| IBIS file stm32l0_71_72_73_81_82_83_wlcsp49.ibs
| Created by s2ibis version 1.1 (customized version)
| North Carolina State University, ERL, 2006
[IBIS ver] 4.2
[File name] stm32l0_71_72_73_81_82_83_wlcsp49.ibs
[File Rev] 1.0
[Date]  14-03-2016
[Source] Data Created at STMicroelectronics
[Notes]  File originated from ELDO simulations.
[Disclaimer]  This information is for modeling purpose only and is
   not guaranted. The information is subject to change without
   notice.
[Copyright] Copyright 2016 STMicroelectronics Inc.
|   Component stm32l0_71_72_73_81_82_83_wlcsp49
[Component] stm32l0_71_72_73_81_82_83_wlcsp49
[Manufacturer] STMicroelectronics
[Package]
| variable   typ   min   max
R_pkg   0.0   0.0   0.0
L_pkg   0.0H   0.0H   0.0H
C_pkg   0.0F   0.0F   0.0F
[Pin]  signal_name   model_name   R_pin   L_pin   C_pin
B6 VLCD POWER
B7 PC13 io8p_wsudq_ls_ft_v33
C6 PC14-OSC32_IN io8p_wsudq_ls_ft_v33
C7 PC15-OSC32_OUT io8p_sudq_ls_tc_esdft
D6 PH0-OSC_IN io8p_sudq_ls_tc_esdft
D7 PH1-OSC_OUT io8p_sudq_ls_tc_esdft
D5 NRST ioreset_ft_v33
C5 PC0 io8p_sudq_lcd4_i2cin_ls_ft
C4 PC1 io8p_sudq_lcd4_i2cin_ls_ft
E7 PC2 io8p_wsudq_lcd4_ls_ft
E6 VREF+ POWER
F7 VDDA POWER
E5 PA0 io8p_wsudq_ls_ft_v33
E4 PA1 io8p_wsudq_lcd4_ls_ft
F6 PA2 io8p_wsudq_lcd4_ls_ft
G7 PA3 io8p_wsudq_lcd4_ls_ft
F5 PA4 io8p_wsudq_i2cin_ls_ft
G6 PA5 io8p_wsudq_i2cin_ls_ft
G5 PA6 io8p_wsudq_lcd4_ls_ft
F4 PA7 io8p_wsudq_lcd4_ls_ft
G4 PB0 io8p_wsudq_lcd4_ls_ft
D3 PB1 io8p_wsudq_lcd4_ls_ft
E3 PB2 io8p_wsudq_lcd4_ls_ft
G3 PB10 io8p_sudq_lcd4_i2cin_ls_ft
F3 PB11 io8p_sudq_lcd4_i2cin_ls_ft
D4 VSS GND
G2 VDD POWER
G1 PB12 io8p_wsudq_lcd4_ls_ft
F2 PB13 io8p_sudq_lcd4_i2cin_ls_ft
F1 PB14 io8p_sudq_lcd4_i2cin_ls_ft
E1 PB15 io8p_wsudq_lcd4_ls_ft
D1 PA8 io8p_sudq_lcd4_i2cin_ls_ft
E2 PA9 io8p_sudq_lcd4_i2cin_ls_ft
C1 PA10 io8p_sudq_lcd4_i2cin_ls_ft
D2 PA11 io8usb_ls_ft
B1 PA12 io8usb_ls_ft
C2 PA13 io8p_sudq_ls_ft
A1 VDD_USB POWER
B2 PA14 io8p_sudq_ls_ft
A2 PA15 io8p_wsudq_lcd4_ls_ft
A3 PB3 io8p_wsudq_lcd4_ls_ft
B3 PB4 io8p_sudq_lcd4_i2cin_ls_ft
A4 PB5 io8p_wsudq_lcd4_ls_ft
B4 PB6 io8p_wsudq_i2cin_ls_ft
C3 PB7 io8p_wsudq_i2cin_ls_ft
A5 BOOT0 vpp_test_hv
B5 PB8 io8p_sudq_lcd4_i2cin_ls_ft
A6 PB9 io8p_sudq_lcd4_i2cin_ls_ft
A7 VDD POWER
[Model Selector] io8p_sudq_ls_ft
io8p00_sudq_ls_ft_pd_lv  "SPEED00 1P8V, PD=40kOhm"
io8p00_sudq_ls_ft_pu_lv  "SPEED00 1P8V, PU=40kOhm"
io8p00_sudq_ls_ft_lv  "SPEED00 1P8V"
io8p01_sudq_ls_ft_pd_lv  "SPEED01 1P8V, PD=40kOhm"
io8p01_sudq_ls_ft_pu_lv  "SPEED01 1P8V, PU=40kOhm"
io8p01_sudq_ls_ft_lv  "SPEED01 1P8V"
io8p10_sudq_ls_ft_pd_lv  "SPEED10 1P8V, PD=40kOhm"
io8p10_sudq_ls_ft_pu_lv  "SPEED10 1P8V, PU=40kOhm"
io8p10_sudq_ls_ft_lv  "SPEED10 1P8V"
io8p11_sudq_ls_ft_pd_lv  "SPEED11 1P8V, PD=40kOhm"
io8p11_sudq_ls_ft_pu_lv  "SPEED11 1P8V, PU=40kOhm"
io8p11_sudq_ls_ft_lv  "SPEED11 1P8V"
io8p00_sudq_ls_ft_pd  "SPEED00, PD=40kOhm"
io8p00_sudq_ls_ft_pu  "SPEED00, PU=40kOhm"
io8p00_sudq_ls_ft  "SPEED00"
io8p01_sudq_ls_ft_pd  "SPEED01, PD=40kOhm"
io8p01_sudq_ls_ft_pu  "SPEED01, PU=40kOhm"
io8p01_sudq_ls_ft  "SPEED01"
io8p10_sudq_ls_ft_pd  "SPEED10, PD=40kOhm"
io8p10_sudq_ls_ft_pu  "SPEED10, PU=40kOhm"
io8p10_sudq_ls_ft  "SPEED10"
io8p11_sudq_ls_ft_pd  "SPEED11, PD=40kOhm"
io8p11_sudq_ls_ft_pu  "SPEED11, PU=40kOhm"
io8p11_sudq_ls_ft  "SPEED11"
[Model Selector] io8p_sudq_ls_tc_esdft
io8p00_sudq_ls_tc_esdft_pd_lv  "SPEED00 1P8V, PD=40kOhm"
io8p00_sudq_ls_tc_esdft_pu_lv  "SPEED00 1P8V, PU=40kOhm"
io8p00_sudq_ls_tc_esdft_lv  "SPEED00 1P8V"
io8p01_sudq_ls_tc_esdft_pd_lv  "SPEED01 1P8V, PD=40kOhm"
io8p01_sudq_ls_tc_esdft_pu_lv  "SPEED01 1P8V, PU=40kOhm"
io8p01_sudq_ls_tc_esdft_lv  "SPEED01 1P8V"
io8p10_sudq_ls_tc_esdft_pd_lv  "SPEED10 1P8V, PD=40kOhm"
io8p10_sudq_ls_tc_esdft_pu_lv  "SPEED10 1P8V, PU=40kOhm"
io8p10_sudq_ls_tc_esdft_lv  "SPEED10 1P8V"
io8p11_sudq_ls_tc_esdft_pd_lv  "SPEED11 1P8V, PD=40kOhm"
io8p11_sudq_ls_tc_esdft_pu_lv  "SPEED11 1P8V, PU=40kOhm"
io8p11_sudq_ls_tc_esdft_lv  "SPEED11 1P8V"
io8p00_sudq_ls_tc_esdft_pd  "SPEED00, PD=40kOhm"
io8p00_sudq_ls_tc_esdft_pu  "SPEED00, PU=40kOhm"
io8p00_sudq_ls_tc_esdft  "SPEED00"
io8p01_sudq_ls_tc_esdft_pd  "SPEED01, PD=40kOhm"
io8p01_sudq_ls_tc_esdft_pu  "SPEED01, PU=40kOhm"
io8p01_sudq_ls_tc_esdft  "SPEED01"
io8p10_sudq_ls_tc_esdft_pd  "SPEED10, PD=40kOhm"
io8p10_sudq_ls_tc_esdft_pu  "SPEED10, PU=40kOhm"
io8p10_sudq_ls_tc_esdft  "SPEED10"
io8p11_sudq_ls_tc_esdft_pd  "SPEED11, PD=40kOhm"
io8p11_sudq_ls_tc_esdft_pu  "SPEED11, PU=40kOhm"
io8p11_sudq_ls_tc_esdft  "SPEED11"
[Model Selector] io8p_wsudq_i2cin_ls_ft
io8p00_wsudq_i2cin_ls_ft_pd_lv  "SPEED00 1P8V, PD=40kOhm"
io8p00_wsudq_i2cin_ls_ft_pu_lv  "SPEED00 1P8V, PU=40kOhm"
io8p00_wsudq_i2cin_ls_ft_lv  "SPEED00 1P8V"
io8p01_wsudq_i2cin_ls_ft_pd_lv  "SPEED01 1P8V, PD=40kOhm"
io8p01_wsudq_i2cin_ls_ft_pu_lv  "SPEED01 1P8V, PU=40kOhm"
io8p01_wsudq_i2cin_ls_ft_lv  "SPEED01 1P8V"
io8p10_wsudq_i2cin_ls_ft_pd_lv  "SPEED10 1P8V, PD=40kOhm"
io8p10_wsudq_i2cin_ls_ft_pu_lv  "SPEED10 1P8V, PU=40kOhm"
io8p10_wsudq_i2cin_ls_ft_lv  "SPEED10 1P8V"
io8p11_wsudq_i2cin_ls_ft_pd_lv  "SPEED11 1P8V, PD=40kOhm"
io8p11_wsudq_i2cin_ls_ft_pu_lv  "SPEED11 1P8V, PU=40kOhm"
io8p11_wsudq_i2cin_ls_ft_lv  "SPEED11 1P8V"
io8p00_wsudq_i2cin_ls_ft_pd  "SPEED00, PD=40kOhm"
io8p00_wsudq_i2cin_ls_ft_pu  "SPEED00, PU=40kOhm"
io8p00_wsudq_i2cin_ls_ft  "SPEED00"
io8p01_wsudq_i2cin_ls_ft_pd  "SPEED01, PD=40kOhm"
io8p01_wsudq_i2cin_ls_ft_pu  "SPEED01, PU=40kOhm"
io8p01_wsudq_i2cin_ls_ft  "SPEED01"
io8p10_wsudq_i2cin_ls_ft_pd  "SPEED10, PD=40kOhm"
io8p10_wsudq_i2cin_ls_ft_pu  "SPEED10, PU=40kOhm"
io8p10_wsudq_i2cin_ls_ft  "SPEED10"
io8p11_wsudq_i2cin_ls_ft_pd  "SPEED11, PD=40kOhm"
io8p11_wsudq_i2cin_ls_ft_pu  "SPEED11, PU=40kOhm"
io8p11_wsudq_i2cin_ls_ft  "SPEED11"
[Model Selector] io8p_wsudq_lcd4_ls_ft
io8p00_wsudq_lcd4_ls_ft_pd_lv  "SPEED00 1P8V, PD=40kOhm"
io8p00_wsudq_lcd4_ls_ft_pu_lv  "SPEED00 1P8V, PU=40kOhm"
io8p00_wsudq_lcd4_ls_ft_lv  "SPEED00 1P8V"
io8p01_wsudq_lcd4_ls_ft_pd_lv  "SPEED01 1P8V, PD=40kOhm"
io8p01_wsudq_lcd4_ls_ft_pu_lv  "SPEED01 1P8V, PU=40kOhm"
io8p01_wsudq_lcd4_ls_ft_lv  "SPEED01 1P8V"
io8p10_wsudq_lcd4_ls_ft_pd_lv  "SPEED10 1P8V, PD=40kOhm"
io8p10_wsudq_lcd4_ls_ft_pu_lv  "SPEED10 1P8V, PU=40kOhm"
io8p10_wsudq_lcd4_ls_ft_lv  "SPEED10 1P8V"
io8p11_wsudq_lcd4_ls_ft_pd_lv  "SPEED11 1P8V, PD=40kOhm"
io8p11_wsudq_lcd4_ls_ft_pu_lv  "SPEED11 1P8V, PU=40kOhm"
io8p11_wsudq_lcd4_ls_ft_lv  "SPEED11 1P8V"
io8p00_wsudq_lcd4_ls_ft_pd  "SPEED00, PD=40kOhm"
io8p00_wsudq_lcd4_ls_ft_pu  "SPEED00, PU=40kOhm"
io8p00_wsudq_lcd4_ls_ft  "SPEED00"
io8p01_wsudq_lcd4_ls_ft_pd  "SPEED01, PD=40kOhm"
io8p01_wsudq_lcd4_ls_ft_pu  "SPEED01, PU=40kOhm"
io8p01_wsudq_lcd4_ls_ft  "SPEED01"
io8p10_wsudq_lcd4_ls_ft_pd  "SPEED10, PD=40kOhm"
io8p10_wsudq_lcd4_ls_ft_pu  "SPEED10, PU=40kOhm"
io8p10_wsudq_lcd4_ls_ft  "SPEED10"
io8p11_wsudq_lcd4_ls_ft_pd  "SPEED11, PD=40kOhm"
io8p11_wsudq_lcd4_ls_ft_pu  "SPEED11, PU=40kOhm"
io8p11_wsudq_lcd4_ls_ft  "SPEED11"
[Model Selector] io8p_wsudq_ls_ft_v33
io8p00_wsudq_ls_ft_v33_pd_lv  "SPEED00 1P8V, PD=40kOhm"
io8p00_wsudq_ls_ft_v33_pu_lv  "SPEED00 1P8V, PU=40kOhm"
io8p00_wsudq_ls_ft_v33_lv  "SPEED00 1P8V"
io8p01_wsudq_ls_ft_v33_pd_lv  "SPEED01 1P8V, PD=40kOhm"
io8p01_wsudq_ls_ft_v33_pu_lv  "SPEED01 1P8V, PU=40kOhm"
io8p01_wsudq_ls_ft_v33_lv  "SPEED01 1P8V"
io8p10_wsudq_ls_ft_v33_pd_lv  "SPEED10 1P8V, PD=40kOhm"
io8p10_wsudq_ls_ft_v33_pu_lv  "SPEED10 1P8V, PU=40kOhm"
io8p10_wsudq_ls_ft_v33_lv  "SPEED10 1P8V"
io8p11_wsudq_ls_ft_v33_pd_lv  "SPEED11 1P8V, PD=40kOhm"
io8p11_wsudq_ls_ft_v33_pu_lv  "SPEED11 1P8V, PU=40kOhm"
io8p11_wsudq_ls_ft_v33_lv  "SPEED11 1P8V"
io8p00_wsudq_ls_ft_v33_pd  "SPEED00, PD=40kOhm"
io8p00_wsudq_ls_ft_v33_pu  "SPEED00, PU=40kOhm"
io8p00_wsudq_ls_ft_v33  "SPEED00"
io8p01_wsudq_ls_ft_v33_pd  "SPEED01, PD=40kOhm"
io8p01_wsudq_ls_ft_v33_pu  "SPEED01, PU=40kOhm"
io8p01_wsudq_ls_ft_v33  "SPEED01"
io8p10_wsudq_ls_ft_v33_pd  "SPEED10, PD=40kOhm"
io8p10_wsudq_ls_ft_v33_pu  "SPEED10, PU=40kOhm"
io8p10_wsudq_ls_ft_v33  "SPEED10"
io8p11_wsudq_ls_ft_v33_pd  "SPEED11, PD=40kOhm"
io8p11_wsudq_ls_ft_v33_pu  "SPEED11, PU=40kOhm"
io8p11_wsudq_ls_ft_v33  "SPEED11"
[Model Selector] vpp_test_hv
vpp_test_hv_2p4  "Input Buffer 1P65V"
vpp_test_hv_3p3  "Input Buffer"
[Model Selector] io8usb_ls_ft
io8usb_ls_ft_dpdn_pu  "HS USB DP/DN IO + PU=1.2kOhm"
io8usb_ls_ft_dpdn  "HS USB DP/DN IO"
io8p00_ls_ft_pd_lv  "SPEED00 1P8V, PD=40kOhm"
io8p00_ls_ft_pu_lv  "SPEED00 1P8V, PU=40kOhm"
io8p00_ls_ft_lv  "SPEED00 1P8V"
io8p01_ls_ft_pd_lv  "SPEED01 1P8V, PD=40kOhm"
io8p01_ls_ft_pu_lv  "SPEED01 1P8V, PU=40kOhm"
io8p01_ls_ft_lv  "SPEED01 1P8V"
io8p10_ls_ft_pd_lv  "SPEED10 1P8V, PD=40kOhm"
io8p10_ls_ft_pu_lv  "SPEED10 1P8V, PU=40kOhm"
io8p10_ls_ft_lv  "SPEED10 1P8V"
io8p11_ls_ft_pd_lv  "SPEED11 1P8V, PD=40kOhm"
io8p11_ls_ft_pu_lv  "SPEED11 1P8V, PU=40kOhm"
io8p11_ls_ft_lv  "SPEED11 1P8V"
io8p00_ls_ft_pd  "SPEED00, PD=40kOhm"
io8p00_ls_ft_pu  "SPEED00, PU=40kOhm"
io8p00_ls_ft  "SPEED00"
io8p01_ls_ft_pd  "SPEED01, PD=40kOhm"
io8p01_ls_ft_pu  "SPEED01, PU=40kOhm"
io8p01_ls_ft  "SPEED01"
io8p10_ls_ft_pd  "SPEED10, PD=40kOhm"
io8p10_ls_ft_pu  "SPEED10, PU=40kOhm"
io8p10_ls_ft  "SPEED10"
io8p11_ls_ft_pd  "SPEED11, PD=40kOhm"
io8p11_ls_ft_pu  "SPEED11, PU=40kOhm"
io8p11_ls_ft  "SPEED11"
[Model Selector] io8p_sudq_lcd4_i2cin_ls_ft
io8p00_sudq_lcd4_i2cin_ls_ft_pd_lv  "SPEED00 1P8V, PD=40kOhm"
io8p00_sudq_lcd4_i2cin_ls_ft_pu_lv  "SPEED00 1P8V, PU=40kOhm"
io8p00_sudq_lcd4_i2cin_ls_ft_lv  "SPEED00 1P8V"
io8p01_sudq_lcd4_i2cin_ls_ft_pd_lv  "SPEED01 1P8V, PD=40kOhm"
io8p01_sudq_lcd4_i2cin_ls_ft_pu_lv  "SPEED01 1P8V, PU=40kOhm"
io8p01_sudq_lcd4_i2cin_ls_ft_lv  "SPEED01 1P8V"
io8p10_sudq_lcd4_i2cin_ls_ft_pd_lv  "SPEED10 1P8V, PD=40kOhm"
io8p10_sudq_lcd4_i2cin_ls_ft_pu_lv  "SPEED10 1P8V, PU=40kOhm"
io8p10_sudq_lcd4_i2cin_ls_ft_lv  "SPEED10 1P8V"
io8p11_sudq_lcd4_i2cin_ls_ft_pd_lv  "SPEED11 1P8V, PD=40kOhm"
io8p11_sudq_lcd4_i2cin_ls_ft_pu_lv  "SPEED11 1P8V, PU=40kOhm"
io8p11_sudq_lcd4_i2cin_ls_ft_lv  "SPEED11 1P8V"
io8p00_sudq_lcd4_i2cin_ls_ft_pd  "SPEED00, PD=40kOhm"
io8p00_sudq_lcd4_i2cin_ls_ft_pu  "SPEED00, PU=40kOhm"
io8p00_sudq_lcd4_i2cin_ls_ft  "SPEED00"
io8p01_sudq_lcd4_i2cin_ls_ft_pd  "SPEED01, PD=40kOhm"
io8p01_sudq_lcd4_i2cin_ls_ft_pu  "SPEED01, PU=40kOhm"
io8p01_sudq_lcd4_i2cin_ls_ft  "SPEED01"
io8p10_sudq_lcd4_i2cin_ls_ft_pd  "SPEED10, PD=40kOhm"
io8p10_sudq_lcd4_i2cin_ls_ft_pu  "SPEED10, PU=40kOhm"
io8p10_sudq_lcd4_i2cin_ls_ft  "SPEED10"
io8p11_sudq_lcd4_i2cin_ls_ft_pd  "SPEED11, PD=40kOhm"
io8p11_sudq_lcd4_i2cin_ls_ft_pu  "SPEED11, PU=40kOhm"
io8p11_sudq_lcd4_i2cin_ls_ft  "SPEED11"
[Model Selector] ioreset_ft_v33
ioreset_ft_v33_pu_lv  "ioreset 1P8V + PU=40kOhm"
ioreset_ft_v33_nopu_lv  "ioreset 1P8V"
ioreset_ft_v33_pu  "ioreset + PU=40kOhm"
ioreset_ft_v33_nopu  "ioreset"
| Models and submodels in the file (176): io8p00_sudq_ls_ft_pd_lv (I/O), io8p00_sudq_ls_ft_pu_lv (I/O), io8p00_sudq_ls_ft_lv (I/O), io8p01_sudq_ls_ft_pd_lv (I/O), io8p01_sudq_ls_ft_pu_lv (I/O), io8p01_sudq_ls_ft_lv (I/O), io8p10_sudq_ls_ft_pd_lv (I/O), io8p10_sudq_ls_ft_pu_lv (I/O), io8p10_sudq_ls_ft_lv (I/O), io8p11_sudq_ls_ft_pd_lv (I/O), io8p11_sudq_ls_ft_pu_lv (I/O), io8p11_sudq_ls_ft_lv (I/O), io8p00_sudq_ls_ft_pd (I/O), io8p00_sudq_ls_ft_pu (I/O), io8p00_sudq_ls_ft (I/O), io8p01_sudq_ls_ft_pd (I/O), io8p01_sudq_ls_ft_pu (I/O), io8p01_sudq_ls_ft (I/O), io8p10_sudq_ls_ft_pd (I/O), io8p10_sudq_ls_ft_pu (I/O), io8p10_sudq_ls_ft (I/O), io8p11_sudq_ls_ft_pd (I/O), io8p11_sudq_ls_ft_pu (I/O), io8p11_sudq_ls_ft (I/O), io8p00_sudq_ls_tc_esdft_pd_lv (I/O), io8p00_sudq_ls_tc_esdft_pu_lv (I/O), io8p00_sudq_ls_tc_esdft_lv (I/O), io8p01_sudq_ls_tc_esdft_pd_lv (I/O), io8p01_sudq_ls_tc_esdft_pu_lv (I/O), io8p01_sudq_ls_tc_esdft_lv (I/O), io8p10_sudq_ls_tc_esdft_pd_lv (I/O), io8p10_sudq_ls_tc_esdft_pu_lv (I/O), io8p10_sudq_ls_tc_esdft_lv (I/O), io8p11_sudq_ls_tc_esdft_pd_lv (I/O), io8p11_sudq_ls_tc_esdft_pu_lv (I/O), io8p11_sudq_ls_tc_esdft_lv (I/O), io8p00_sudq_ls_tc_esdft_pd (I/O), io8p00_sudq_ls_tc_esdft_pu (I/O), io8p00_sudq_ls_tc_esdft (I/O), io8p01_sudq_ls_tc_esdft_pd (I/O), io8p01_sudq_ls_tc_esdft_pu (I/O), io8p01_sudq_ls_tc_esdft (I/O), io8p10_sudq_ls_tc_esdft_pd (I/O), io8p10_sudq_ls_tc_esdft_pu (I/O), io8p10_sudq_ls_tc_esdft (I/O), io8p11_sudq_ls_tc_esdft_pd (I/O), io8p11_sudq_ls_tc_esdft_pu (I/O), io8p11_sudq_ls_tc_esdft (I/O), io8p00_wsudq_i2cin_ls_ft_pd_lv (I/O), io8p00_wsudq_i2cin_ls_ft_pu_lv (I/O), io8p00_wsudq_i2cin_ls_ft_lv (I/O), io8p01_wsudq_i2cin_ls_ft_pd_lv (I/O), io8p01_wsudq_i2cin_ls_ft_pu_lv (I/O), io8p01_wsudq_i2cin_ls_ft_lv (I/O), io8p10_wsudq_i2cin_ls_ft_pd_lv (I/O), io8p10_wsudq_i2cin_ls_ft_pu_lv (I/O), io8p10_wsudq_i2cin_ls_ft_lv (I/O), io8p11_wsudq_i2cin_ls_ft_pd_lv (I/O), io8p11_wsudq_i2cin_ls_ft_pu_lv (I/O), io8p11_wsudq_i2cin_ls_ft_lv (I/O), io8p00_wsudq_i2cin_ls_ft_pd (I/O), io8p00_wsudq_i2cin_ls_ft_pu (I/O), io8p00_wsudq_i2cin_ls_ft (I/O), io8p01_wsudq_i2cin_ls_ft_pd (I/O), io8p01_wsudq_i2cin_ls_ft_pu (I/O), io8p01_wsudq_i2cin_ls_ft (I/O), io8p10_wsudq_i2cin_ls_ft_pd (I/O), io8p10_wsudq_i2cin_ls_ft_pu (I/O), io8p10_wsudq_i2cin_ls_ft (I/O), io8p11_wsudq_i2cin_ls_ft_pd (I/O), io8p11_wsudq_i2cin_ls_ft_pu (I/O), io8p11_wsudq_i2cin_ls_ft (I/O), io8p00_wsudq_lcd4_ls_ft_pd_lv (I/O), io8p00_wsudq_lcd4_ls_ft_pu_lv (I/O), io8p00_wsudq_lcd4_ls_ft_lv (I/O), io8p01_wsudq_lcd4_ls_ft_pd_lv (I/O), io8p01_wsudq_lcd4_ls_ft_pu_lv (I/O), io8p01_wsudq_lcd4_ls_ft_lv (I/O), io8p10_wsudq_lcd4_ls_ft_pd_lv (I/O), io8p10_wsudq_lcd4_ls_ft_pu_lv (I/O)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
